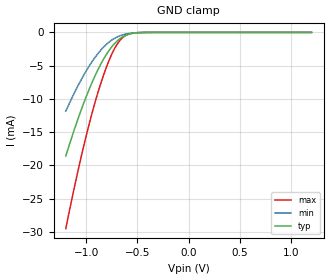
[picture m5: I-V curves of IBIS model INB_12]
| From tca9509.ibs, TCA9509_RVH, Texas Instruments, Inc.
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[Model]   INB_12
Model_type  Input
Vinl=0.15
Vinh=0.84
| variable   typ   min   max
C_comp   1.54pF   1.06pF   1.77pF
[Temperature Range]   40   100   -40
| Ambient temperature   25   85   -40
[Voltage range]   1.2   1.1   1.3
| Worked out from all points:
|   GND clamp passes 1 mA (typ) near -0.68 V on its own axis
[GND Clamp]
| INB_12
|   Voltage   I(typ)   I(min)   I(max)
-1.2V     -18.61mA   -11.86mA   -29.54mA
-1.12V    -14.77mA   -9.228mA   -23.57mA
-1.04V    -11.26mA   -6.859mA   -18.07mA
-965mV    -8.314mA   -4.909mA   -13.39mA
-890mV    -5.741mA   -3.265mA   -9.247mA
-820mV    -3.73mA    -2.044mA   -5.935mA
-755mV    -2.25mA    -1.202mA   -3.417mA
-695mV    -1.248mA   -666.5uA   -1.7mA
-640mV    -634.6uA   -353.3uA   -732.1uA
-570mV    -213.8uA   -137.7uA   -186.4uA
-465mV    -28.41uA   -25.44uA   -14.85uA
1.2V      155.6pA    881.8pA    20.05pA
